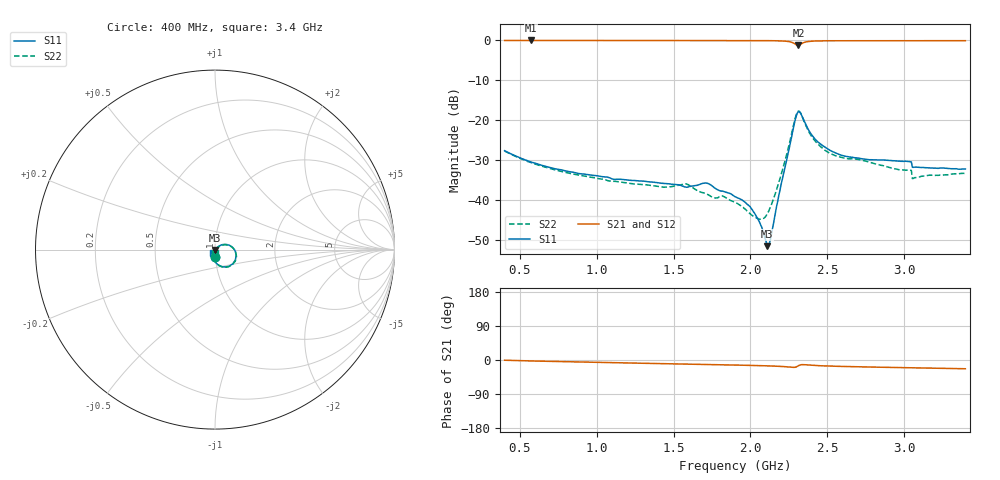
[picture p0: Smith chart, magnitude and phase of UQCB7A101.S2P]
!  Part Number  UQCB7A101	Mounting Orientation: Vertical
!  Description: RF capacitors
!  Application: Coupling, Bypass, Tuning, DC Block
!  Filters, Matching
# GHZ S DB R 50
! Freq  |S11|  S11 Ph  |S21|  S21 Ph  |S12|  S12 Ph  |S22|  S22 Ph
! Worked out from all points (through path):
!   401 points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, 400 MHz to 3.4 GHz, reference 50 ohm
!   highest |S21| = -0.03 dB at 573 MHz (marker M1); lowest = -1.2 dB at 2.313 GHz (marker M2)
!   group delay of S21, straight-line fit = 19.7 ps
!   lowest |S11| = -51.6 dB at 2.11 GHz (marker M3), VSWR 1.01, Z = 50.2 - j0.175 ohm
!   |S11| at or under -10 dB: start of sweep to end of sweep
!   |S22| runs from -44.8 to -17.7 dB; largest |S21 - S12| = 0.0024
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0.4  -27.67 -87.6  -0.03 -0.6  -0.02 -0.6  -27.74 -87.9
0.573  -30.51 -87.8  -0.03 -2.5  -0.02 -2.5  -30.66 -88.0
0.903  -33.48 -88.7  -0.04 -5.5  -0.03 -5.5  -33.91 -87.7
1.405  -35.74 -93.3  -0.05 -9.4  -0.04 -9.4  -36.67 -85.6
1.578  -36.79 -93.8  -0.06 -10.8  -0.05 -10.8  -35.99 -87.5
1.713  -35.78 -96.7  -0.06 -11.8  -0.05 -11.8  -38.52 -90.4
1.9  -39.19 -100.7  -0.06 -13.3  -0.05 -13.3  -40.57 -80.1
2.013  -42.51 -97.1  -0.07 -14.3  -0.06 -14.4  -43.92 -60.2
2.073  -46.74 -81.5  -0.08 -15.0  -0.07 -15.0  -44.84 -28.9
2.11  -51.60 -41.6  -0.08 -15.4  -0.07 -15.5  -43.50 -1.2
2.133  -49.56 5.2  -0.09 -15.8  -0.08 -15.8  -41.64 12.6
2.208  -34.88 43.5  -0.16 -17.2  -0.14 -17.2  -32.66 34.9
2.275  -22.92 23.5  -0.58 -19.4  -0.57 -19.4  -22.27 18.5
2.298  -19.08 -2.2  -1.08 -18.4  -1.07 -18.5  -18.74 -6.0
2.313  -17.89 -26.9  -1.23 -15.2  -1.22 -15.3  -17.72 -30.0
2.403  -23.88 -91.2  -0.21 -14.1  -0.19 -14.1  -24.30 -90.5
2.485  -26.77 -100.7  -0.12 -15.6  -0.11 -15.7  -27.55 -97.7
2.59  -28.78 -104.1  -0.11 -16.9  -0.09 -16.9  -29.34 -98.5
2.905  -30.11 -108.0  -0.11 -19.6  -0.10 -19.6  -31.87 -108.3
3.033  -30.39 -111.2  -0.13 -20.3  -0.12 -20.4  -32.53 -106.8
3.07  -31.79 -111.2  -0.12 -20.6  -0.11 -20.6  -34.42 -89.5
3.4  -32.27 -122.8  -0.09 -23.1  -0.08 -23.1  -33.37 -95.1
